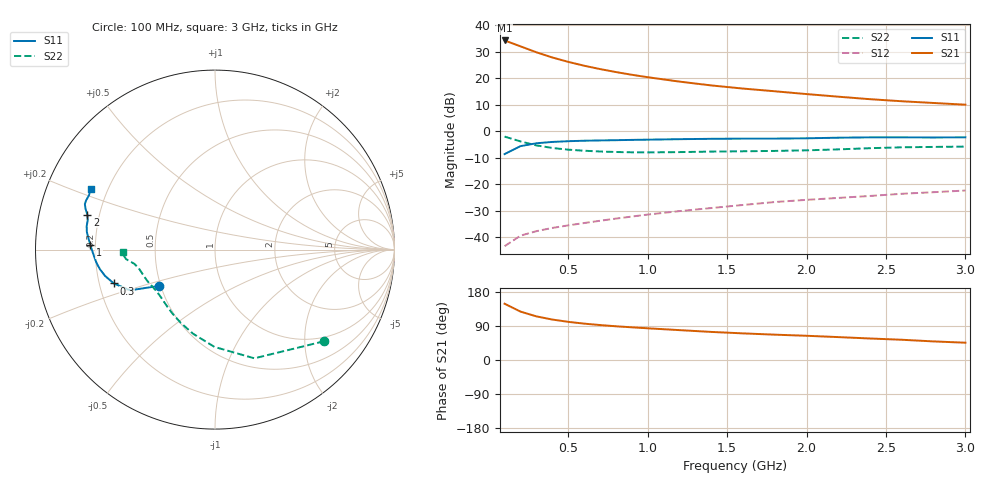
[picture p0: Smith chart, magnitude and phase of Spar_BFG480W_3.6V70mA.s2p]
! Filename: 3_670BFG480.001
! Title: BFG480W
! Bias: Vce=3.6V; Ic=70mA
! Company: NXP Semiconductors NL
! User: Quality&Reliability T&D
! Measure time: 10 Nov 1999 / 12:00:21
#  MHz  S  MA  R 50
! Freq  S11  S21  S12  S22  :
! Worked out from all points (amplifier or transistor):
!   20 points, 100 MHz to 3 GHz, reference 50 ohm
!   highest |S21| = 34.3 dB at 100 MHz (marker M1)
!   |S21| within 3 dB of that: start of sweep to 234.7 MHz
!   unconditionally stable (mu >= 1): 838.9 MHz to end of sweep
!   at 400 MHz: K = 0.73, MSG = 32.2 dB, |S12| = -36.5 dB
!   at 1.2 GHz: K = 1.06, MAG = 22.9 dB, |S12| = -30.1 dB
!   at 3 GHz: K = 1.05, MAG = 14.8 dB, |S12| = -22.3 dB
!   S11 on the Smith chart (normalised r, x): 100 MHz: 0.49, -0.23; 300 MHz: 0.26, -0.15; 1 GHz: 0.18, +0.02; 2 GHz: 0.15, +0.13; 3 GHz: 0.14, +0.23
100  0.3719 -147.0  51.68 148.5  0.006805 68.7  0.7939 -40.0
200  0.5244 -154.4  40.01 127.7  0.01076 59.2  0.6442 -70.1
300  0.5943 -161.5  30.92 115.1  0.01306 56.9  0.5421 -90.3
400  0.6296 -166.5  24.69 106.8  0.01502 57.4  0.4843 -104.6
500  0.6502 -170.3  20.4 100.7  0.01678 59.0  0.4503 -115.1
600  0.6632 -173.3  17.26 96.0  0.01859 60.9  0.4296 -123.0
700  0.672 -175.9  14.93 92.2  0.02051 62.9  0.4157 -129.2
800  0.6794 -178.2  13.11 89.0  0.02253 65.0  0.4065 -134.4
900  0.6877 179.7  11.65 86.3  0.02461 66.9  0.4013 -138.8
1000  0.6947 177.8  10.48 83.7  0.02684 68.2  0.3997 -142.8
1200  0.7099 174.6  8.655 78.8  0.03118 70.3  0.4048 -149.3
1400  0.7208 172.1  7.331 74.1  0.03565 71.6  0.4139 -154.1
1600  0.7268 169.7  6.395 70.2  0.04074 72.8  0.4196 -157.8
1800  0.7278 167.0  5.687 66.9  0.04627 73.6  0.4263 -161.6
2000  0.7373 164.7  5.035 63.9  0.0509 74.5  0.437 -166.1
2200  0.7565 162.5  4.493 60.4  0.05535 74.6  0.4558 -169.9
2400  0.7682 160.7  4.03 56.7  0.06025 74.2  0.4798 -172.3
2600  0.7687 159.0  3.685 53.4  0.06623 73.7  0.4986 -173.9
2800  0.7646 156.8  3.418 49.0  0.07095 72.5  0.5072 -175.8
3000  0.7695 154.1  3.174 45.6  0.07632 71.8  0.5146 -178.7
